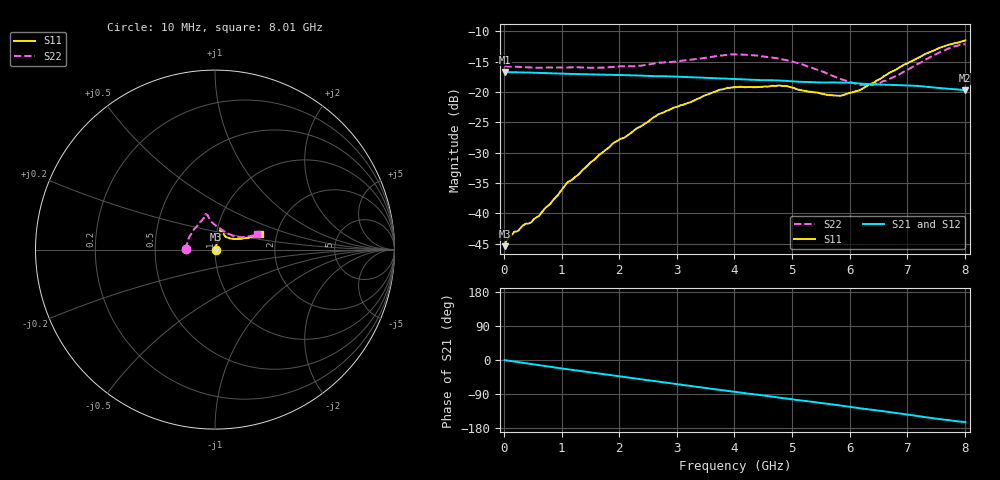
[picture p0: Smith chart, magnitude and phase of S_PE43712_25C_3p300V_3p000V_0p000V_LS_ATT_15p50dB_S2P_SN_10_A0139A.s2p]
! DEVICE ID: PE43712
! File Path: z:\PE43713\PE43713_CHAR_NOM_04292014\AMB\3p300\LS_ATT_15p50dB\PE43713_AMB_3p300V_3p000V_0p000V_LS_ATT_15p50dB_S2P_SN_10_A0139A.s2p
! Serial: 10
! Lot: A0139A
! Temp: 25C
! VDD: 3.300
! VSS: 0.000
! Control_Hi: 3.000
! Control_Lo: 0.000
! Attenuation Step: 15.50dB
! Port 1: RF1
! Port 2: RF2
! ThroughPath:1-2
! IDD: 0.000147515
! ISS: -9.22e-008
#  Hz  S  RI  R  50
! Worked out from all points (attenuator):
!   801 points, 10 MHz to 8.01 GHz, reference 50 ohm
!   highest |S21| = -16.71 dB at 10 MHz (marker M1); lowest = -19.7 dB at 8 GHz (marker M2)
!   lowest |S11| = -45.4 dB at 10 MHz (marker M3), VSWR 1.01, Z = 50.5 + j0.0424 ohm
!   |S11| at or under -10 dB: start of sweep to end of sweep
!   |S22| runs from -18.9 to -12.1 dB; largest |S21 - S12| = 0.00053
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1e7  0.00533 0.000419  0.1461 -0.000751  0.1462 -0.000728  -0.1635 0.00114
1.6e8  0.00644 0.00236  0.1453 -0.00966  0.1454 -0.00965  -0.1613 0.0113
6.1e8  0.00597 0.00744  0.1395 -0.0345  0.1395 -0.0345  -0.1542 0.0365
9.2e8  0.00508 0.0129  0.1331 -0.05  0.1332 -0.05  -0.1499 0.054
1.09e9  0.00509 0.017  0.1289 -0.0578  0.129 -0.0579  -0.1457 0.0642
1.35e9  0.00605 0.0216  0.1222 -0.0691  0.1222 -0.0691  -0.1392 0.0772
1.9e9  0.0117 0.0361  0.1047 -0.0905  0.1047 -0.0904  -0.1196 0.1086
2.34e9  0.0185 0.0476  0.0879 -0.1048  0.0878 -0.1048  -0.1008 0.1296
2.68e9  0.0256 0.0604  0.0737 -0.1129  0.0737 -0.1129  -0.0848 0.1525
3.72e9  0.0321 0.0981  0.0264 -0.1268  0.0263 -0.1268  -0.0558 0.1905
4.01e9  0.0321 0.1048  0.0132 -0.1274  0.0132 -0.1273  -0.0538 0.1973
4.79e9  0.0327 0.1084  -0.0205 -0.1224  -0.0205 -0.1225  -0.0383 0.184
5.35e9  0.0438 0.0897  -0.0419 -0.1132  -0.0419 -0.1131  -0.0218 0.1567
5.87e9  0.0638 0.0686  -0.0608 -0.103  -0.0608 -0.1029  0.016 0.1259
6.16e9  0.0816 0.0627  -0.0708 -0.0938  -0.0706 -0.0939  0.0442 0.1063
6.29e9  0.0932 0.0606  -0.0739 -0.09  -0.0737 -0.09  0.0589 0.0972
6.42e9  0.1034 0.0599  -0.0772 -0.0863  -0.077 -0.0863  0.0731 0.0885
6.68e9  0.1298 0.0597  -0.0839 -0.078  -0.0837 -0.078  0.1026 0.0756
7.37e9  0.1994 0.0704  -0.0971 -0.0516  -0.097 -0.0516  0.1764 0.0718
7.71e9  0.2312 0.0789  -0.099 -0.0389  -0.099 -0.039  0.2138 0.0795
8e9  0.25 0.089  -0.0993 -0.0286  -0.0992 -0.0288  0.233 0.0843
8.01e9  0.2506 0.0897  -0.0994 -0.0284  -0.0992 -0.0286  0.2336 0.0842
